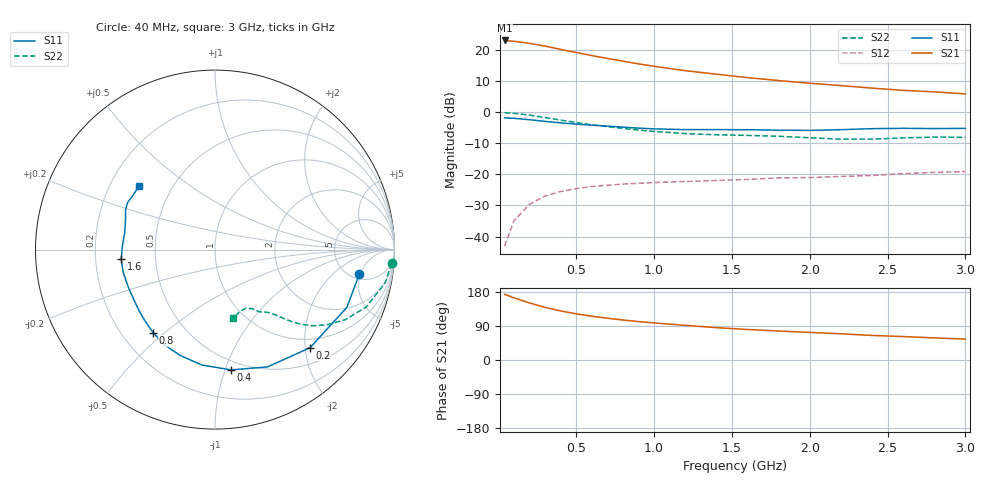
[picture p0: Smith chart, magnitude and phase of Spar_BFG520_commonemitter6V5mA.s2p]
! Filename:  BFG520H.S2P  Version:  2.1
! NXP part #: BFG520  Date: Feb 1992
! Bias condition: Vce=6V, Ic=5mA
! IN LINE PINNING: same data as with cross emitter pinning.
#  MHz  S  MA  R  50
! Freq  S11  S21  S12  S22  !GUM [dB]
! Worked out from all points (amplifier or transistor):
!   21 points, 40 MHz to 3 GHz, reference 50 ohm
!   highest |S21| = 23.2 dB at 40 MHz (marker M1)
!   |S21| within 3 dB of that: start of sweep to 411.7 MHz
!   unconditionally stable (mu >= 1): 1.807 GHz to end of sweep
!   at 300 MHz: K = 0.19, MSG = 24.1 dB, |S12| = -26.9 dB
!   at 1 GHz: K = 0.63, MSG = 18.7 dB, |S12| = -22.6 dB
!   at 3 GHz: K = 1.29, MAG = 9.3 dB, |S12| = -19.1 dB
!   lowest NFmin = 0.90 dB at 500 MHz
!   S11 on the Smith chart (normalised r, x): 40 MHz: 5.89, -4.80; 200 MHz: 0.81, -2.10; 400 MHz: 0.42, -1.05; 800 MHz: 0.33, -0.46; 1.6 GHz: 0.31, -0.04; 3 GHz: 0.32, +0.33
40  0.816 -9.6  14.37 173.3  0.007 84.3  0.987 -4.5
100  0.802 -23.7  13.95 164.2  0.018 78.1  0.966 -11.1
200  0.761 -45.9  12.88 150.6  0.033 67.3  0.901 -20.8
300  0.716 -65.9  11.66 138.8  0.045 59.2  0.824 -28.3
400  0.676 -82.4  10.31 129.5  0.053 53.4  0.75 -34.0
500  0.647 -96.6  9.188 121.9  0.059 48.8  0.686 -38.2
600  0.621 -108.1  8.202 115.5  0.064 45.8  0.632 -41.1
700  0.601 -117.8  7.379 110.3  0.067 43.2  0.587 -43.1
800  0.577 -126.6  6.665 105.5  0.07 42.3  0.552 -44.7
900  0.557 -134.5  6.028 101.3  0.072 41.6  0.519 -46.0
1000  0.542 -141.8  5.513 97.9  0.074 41.4  0.493 -47.3
1200  0.527 -155.4  4.695 91.4  0.077 41.0  0.455 -50.1
1400  0.527 -166.0  4.116 85.4  0.08 41.1  0.435 -53.0
1600  0.525 -174.4  3.623 80.5  0.083 43.3  0.425 -54.6
1800  0.516 177.5  3.25 76.5  0.088 44.6  0.412 -55.8
2000  0.512 169.1  2.941 72.8  0.089 46.6  0.39 -57.6
2200  0.526 161.4  2.695 69.2  0.093 47.4  0.37 -62.1
2400  0.546 155.8  2.454 64.8  0.096 49.9  0.37 -68.0
2600  0.553 151.7  2.259 61.9  0.103 51.8  0.387 -72.5
2800  0.548 146.7  2.138 58.3  0.108 52.2  0.4 -74.2
3000  0.552 140.3  1.982 55.1  0.111 54.5  0.395 -75.4
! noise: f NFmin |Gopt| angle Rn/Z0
500  0.9  0.439  29  0.27
900  1.1  0.395  49  0.28
1000  1.15  0.4  53  0.29
2000  1.85  0.312  126  0.17
